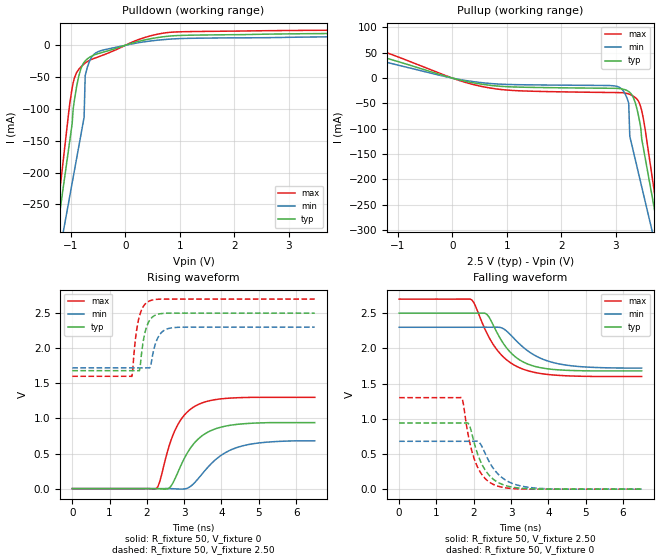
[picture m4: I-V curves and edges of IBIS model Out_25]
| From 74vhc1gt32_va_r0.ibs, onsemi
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|//////////////////////////////////////////////////////////////////////////////
|//////////////////////////////////////////////////////////////////////////////
[Model] Out_25
Model_type Output
Polarity Non-Inverting
Vmeas = 1.25
Vref = 2.50
Rref = 1k
Cref = 15pF
|  variable   typ   min   max
C_comp   3.9pF   3.9pF   3.9pF
|//////////////////////////////////////////////////////////////////////////////
[Temperature Range]   25   125   -55
|//////////////////////////////////////////////////////////////////////////////
[Voltage Range]   2.50V   2.30V   2.70V
|//////////////////////////////////////////////////////////////////////////////
[Pulldown Reference]   0V   0V   0V
|//////////////////////////////////////////////////////////////////////////////
[Pullup Reference]   2.50V   2.30V   2.70V
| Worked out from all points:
|   slope of the pulldown table from 0 to 0.375 V, typ, clamps not added: 43 ohm
|   slope of the pullup table from 0 to 0.375 V, typ, clamps not added: 41 ohm
|   falling waveform, R_fixture 50, V_fixture 2.50: 20-80 % time 690ps typ, 899ps min, 784ps max; typ from 2.5 V to 1.68 V
|   falling waveform, R_fixture 50, V_fixture 0: 20-80 % time 462ps typ, 558ps min, 387ps max; typ from 0.94 V to 0 V
|   rising waveform, R_fixture 50, V_fixture 0: 20-80 % time 684ps typ, 854ps min, 571ps max; typ from 0 V to 0.94 V
|   rising waveform, R_fixture 50, V_fixture 2.50: 20-80 % time 175ps typ, 200ps min, 174ps max; typ from 1.68 V to 2.5 V
|//////////////////////////////////////////////////////////////////////////////
[Pulldown]
|   Voltage   I(typ)   I(min)   I(max)
-2.5V     -1.071A    -926.6mA   -1.221A
-1.38V    -368mA     -404.3mA   -358.8mA
-1.26V    -294.7mA   -348.1mA   -268.4mA
-1.12V    -209.2mA   -282.3mA   -163.4mA
-980mV    -123.4mA   -216.5mA   -67.25mA
-960mV    -99.63mA   -207.1mA   -58.62mA
-860mV    -49.15mA   -160.1mA   -37.95mA
-760mV    -26.68mA   -113mA     -29.31mA
-740mV    -24.56mA   -47.71mA   -27.94mA
-500mV    -13.1mA    -9.923mA   -18.28mA
820mV     14.46mA    9.667mA    20.31mA
5V        19.19mA    14.05mA    24.34mA
|//////////////////////////////////////////////////////////////////////////////
[Pullup]
|   Voltage   I(typ)   I(min)   I(max)
-2.5V     78.63mA    63.73mA    97.94mA
500mV     -11.48mA   -8.594mA   -15.68mA
3.06V     -20.62mA   -17.92mA   -28.7mA
3.24V     -26.57mA   -50.02mA   -31.48mA
3.26V     -28.29mA   -115mA     -32.32mA
3.36V     -48.75mA   -160.6mA   -38.46mA
3.46V     -97.3mA    -206.2mA   -56.84mA
3.48V     -120.7mA   -215.4mA   -65.04mA
3.64V     -215.8mA   -288.3mA   -173mA
3.76V     -287.1mA   -343mA     -260.5mA
3.84V     -334.7mA   -379.5mA   -318.8mA
5V        -1.024A    -908.6mA   -1.165A
|//////////////////////////////////////////////////////////////////////////////
|//////////////////////////////////////////////////////////////////////////////
[Ramp]
|  variable   typ   min   max
dV/dt_r   5.640E-01/7.000E-10  4.080E-01/8.500E-10  7.800E-01/5.500E-10
dV/dt_f   4.920E-01/7.000E-10  3.480E-01/9.000E-10  6.600E-01/8.000E-10
R_load = 50
|/////////////////////////////////////////////////////////////////////////////
[Falling Waveform]
R_fixture = 50
V_fixture = 2.50
V_fixture_min = 2.30
V_fixture_max = 2.70
C_fixture = 0p
|   time   V(typ)   V(min)   V(max)
0s        2.5V       2.3V       2.7V
1.95ns    2.5V       2.3V       2.689V
2.35ns    2.484V     2.3V       2.217V
2.6ns     2.248V     2.301V     1.996V
2.75ns    2.105V     2.291V     1.901V
2.95ns    1.963V     2.211V     1.809V
3.4ns     1.788V     1.984V     1.69V
3.85ns    1.72V      1.847V     1.639V
4.4ns     1.691V     1.768V     1.613V
6.5ns     1.68V      1.72V      1.6V
|//////////////////////////////////////////////////////////////////////////////
[Falling Waveform]
R_fixture = 50
V_fixture = 0
C_fixture = 0p
|   time   V(typ)   V(min)   V(max)
0s        940mV      680mV      1.3V
1.675ns   939.9mV    680mV      1.299V
1.725ns   939.5mV    680mV      1.2V
1.875ns   917.4mV    679.7mV    705.9mV
2.05ns    586.5mV    682.2mV    377.8mV
2.3ns     276.5mV    514.7mV    153.9mV
2.6ns     111.8mV    244.2mV    51.1mV
2.95ns    37.84mV    101mV      12.56mV
3.5ns     5.237mV    24.03mV    0V
6.5ns     0V         0V         0V
|//////////////////////////////////////////////////////////////////////////////
[Rising Waveform]
R_fixture = 50
V_fixture = 0
C_fixture = 0p
|   time   V(typ)   V(min)   V(max)
0s        0V         0V         0V
2.25ns    1.112mV    -3.687uV   -2.148mV
2.35ns    -2.202mV   16.23uV    108.9mV
2.6ns     9.092mV    668uV      614.3mV
2.8ns     194.5mV    -4.556mV   881.8mV
3.1ns     522.2mV    9.309mV    1.1V
3.45ns    740.4mV    189.3mV    1.215V
3.95ns    870.3mV    458.8mV    1.276V
4.45ns    917mV      591.4mV    1.295V
6.5ns     940mV      680mV      1.3V
|//////////////////////////////////////////////////////////////////////////////
[Rising Waveform]
R_fixture = 50
V_fixture = 2.50
V_fixture_min = 2.30
V_fixture_max = 2.70
C_fixture = 0p
|   time   V(typ)   V(min)   V(max)
0s        1.68V      1.72V      1.6V
1.6ns     1.68V      1.72V      1.599V
1.7ns     1.68V      1.72V      2.159V
1.775ns   1.68V      1.72V      2.402V
1.8ns     1.678V     1.72V      2.456V
1.95ns    2.225V     1.72V      2.627V
2.1ns     2.417V     1.737V     2.679V
2.3ns     2.484V     2.155V     2.697V
2.6ns     2.5V       2.283V     2.7V
6.5ns     2.5V       2.3V       2.7V
